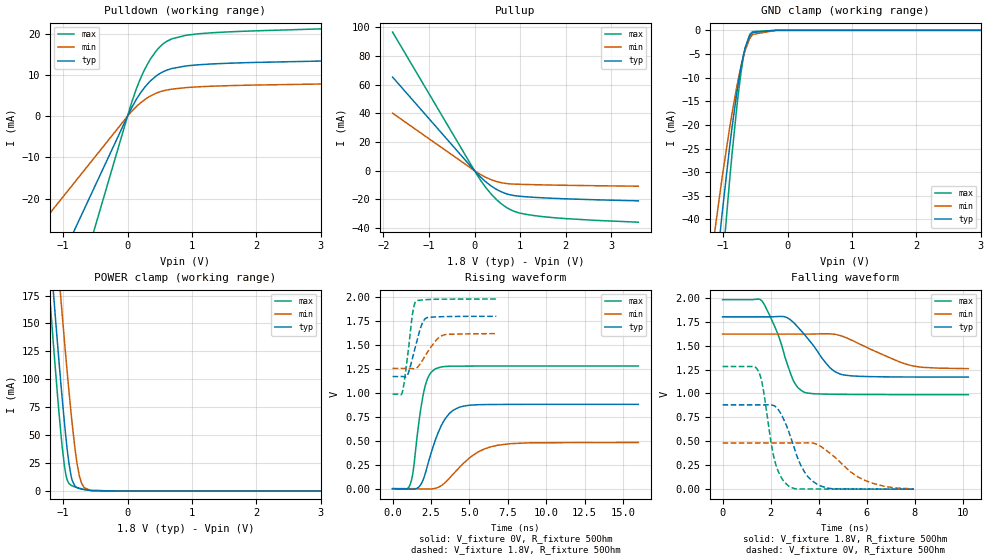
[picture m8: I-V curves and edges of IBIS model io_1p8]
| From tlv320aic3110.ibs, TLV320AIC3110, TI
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|   io_1p8 Model
[Model]   io_1p8
Model_type   I/O
Polarity   Non-Inverting
Enable   Active-High
Vinl = 0.54
Vinh = 1.26
Vmeas = 0.9
Vref = 0
Cref = 10pF
Rref = 100
|   typ   min   max
|   (nom PVT)   (fast PVT)   (slow PVT)
C_comp   1.467e-12   1.439e-12   1.494e-12
| Where nom  PVT is Nominal Process, 1.8V, 27C
|   Fast PVT is Strong Process,  1.98V, -40C
|   Slow PVT is Weak Process,   1.62V, 125C
[Model spec]
Vinl   0.54   0.486   0.594
Vinh   1.26   1.134   1.386
[Voltage Range]   1.8   1.62   1.98
|Junction Temperature
[Temperature Range]   27   125   -40
[Pullup Reference]   1.8   1.62   1.98
[Pulldown Reference]   0   0   0
[Power Clamp Reference]   1.8   1.62   1.98
[GND Clamp Reference]   0   0   0
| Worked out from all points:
|   slope of the pulldown table from 0 to 0.27 V, typ, clamps not added: 38.1 ohm
|   slope of the pullup table from 0 to 0.27 V, typ, clamps not added: 32.3 ohm
|   GND clamp passes 1 mA (typ) near -0.58 V on its own axis
|   POWER clamp passes 1 mA (typ) near -0.65 V on its own axis
|   falling waveform, V_fixture 1.8V, R_fixture 50Ohm: 20-80 % time 1.17ns typ, 1.9ns min, 842ps max; typ from 1.8 V to 1.17 V
|   rising waveform, V_fixture 0V, R_fixture 50Ohm: 20-80 % time 1.17ns typ, 1.99ns min, 651ps max; typ from 0 V to 0.881 V
|   rising waveform, V_fixture 1.8V, R_fixture 50Ohm: 20-80 % time 624ps typ, 920ps min, 442ps max; typ from 1.17 V to 1.8 V
|   falling waveform, V_fixture 0V, R_fixture 50Ohm: 20-80 % time 831ps typ, 1.46ns min, 513ps max; typ from 0.881 V to 0 V
[Pulldown]
|   Voltage   I(typ)   I(min)   I(max)
-1.8V     -60.44mA   -35.18mA   -96.09mA
-85.32mV  -2.865mA   -1.668mA   -4.555mA
67.86mV   2.164mA    1.237mA    3.517mA
173.2mV   5mA        2.868mA    8.101mA
252.5mV   6.752mA    3.877mA    10.93mA
356.2mV   8.586mA    4.927mA    13.91mA
443.3mV   9.762mA    5.588mA    15.84mA
605.7mV   11.18mA    6.359mA    18.17mA
688.9mV   11.6mA     6.589mA    18.81mA
898.9mV   12.2mA     6.948mA    19.65mA
1.307V    12.71mA    7.299mA    20.29mA
3.598V    13.69mA    8.018mA    21.69mA
[GND Clamp]
|   Voltage   I(typ)   I(min)   I(max)
-1.8V     -228.8mA   -131.4mA   -346.6mA
-1.18V    -60.79mA   -47.45mA   -78.73mA
-1.018V   -38.93mA   -31.27mA   -50.57mA
-898.2mV  -24.52mA   -20.52mA   -31.5mA
-783mV    -12.73mA   -11.53mA   -15.61mA
-736.7mV  -8.832mA   -8.46mA    -10.36mA
-685.8mV  -5.288mA   -5.563mA   -5.688mA
-657.5mV  -3.723mA   -4.215mA   -3.718mA
-588.2mV  -1.211mA   -1.797mA   -915uA
-541.8mV  -455.1uA   -870.4uA   -271.3uA
-180mV    0A         -194.6nA   0A
3.598V    0A         0A         0A
[Pullup]
|   Voltage   I(typ)   I(min)   I(max)
-1.8V     65.35mA    40.15mA    96.77mA
67.14mV   -2.325mA   -1.411mA   -3.476mA
207.7mV   -6.661mA   -3.989mA   -10.05mA
360mV     -10.54mA   -6.205mA   -16.11mA
591.8mV   -14.82mA   -8.42mA    -23.2mA
720.7mV   -16.34mA   -9.058mA   -26.04mA
898.9mV   -17.53mA   -9.423mA   -28.71mA
1.331V    -18.66mA   -9.804mA   -31.46mA
1.981V    -19.63mA   -10.2mA    -33.43mA
3.598V    -21.07mA   -10.85mA   -35.98mA
[POWER Clamp]
|   Voltage   I(typ)   I(min)   I(max)
-1.8V     683mA      751.1mA    650.3mA
-1.215V   224.9mA    301.8mA    179.4mA
-1.184V   202.1mA    279.2mA    156.2mA
-1.137V   167.6mA    244.9mA    121.2mA
-1.032V   94.01mA    170mA      49.48mA
-959.4mV  49.04mA    120.9mA    15.03mA
-876.6mV  13.34mA    69.64mA    5.038mA
-816.7mV  4.338mA    38.31mA    3.606mA
-747mV    2.078mA    13.26mA    2.384mA
-674.1mV  1.18mA     3.013mA    1.351mA
-578.3mV  431.7uA    544.6uA    424.2uA
3.598V    0A         0A         0A
[Ramp]
R_load = 50
|   typ   min   max
dV/dt_r   0.52844/1.16363e-09   0.289575/1.9791e-09   0.768595/6.51078e-10
dV/dt_f   0.377553/1.16602e-09   0.217999/1.91494e-09   0.595446/8.39797e-10
[Falling Waveform]
V_fixture = 1.8V
V_fixture_min = 1.62V
V_fixture_max = 1.98V
R_fixture = 50Ohm
|   Time   V(typ)   V(min)   V(max)
0s        1.8V       1.62V      1.98V
1.634ns   1.8V       1.62V      1.968V
2.288ns   1.804V     1.62V      1.629V
2.672ns   1.794V     1.62V      1.323V
2.927ns   1.747V     1.62V      1.145V
3.383ns   1.623V     1.62V      1.015V
4.456ns   1.272V     1.623V     992mV
4.941ns   1.199V     1.601V     990.4mV
7.836ns   1.172V     1.292V     987.8mV
10.23ns   1.171V     1.259V     987.6mV
[Rising Waveform]
V_fixture = 0V
V_fixture_min = 0V
V_fixture_max = 0V
R_fixture = 50Ohm
|   Time   V(typ)   V(min)   V(max)
0s        982.6pV    22.07nV    579.6pV
1.163ns   -4.767mV   75.04uV    51.74mV
1.352ns   -5.16mV    326.5uV    193.8mV
1.754ns   25.18mV    -2.679mV   741.6mV
2.05ns    117.8mV    -3.762mV   1.024V
2.802ns   514.5mV    4.754mV    1.252V
3.984ns   822.4mV    158.7mV    1.279V
5.239ns   874mV      349.2mV    1.28V
6.822ns   879.4mV    452.9mV    1.281V
16ns      880.7mV    482.6mV    1.281V
[Rising Waveform]
V_fixture = 1.8V
V_fixture_min = 1.62V
V_fixture_max = 1.98V
R_fixture = 50Ohm
|   Time   V(typ)   V(min)   V(max)
0s        1.171V     1.257V     987.6mV
643ps     1.171V     1.257V     1.011V
949ps     1.179V     1.257V     1.346V
1.308ns   1.371V     1.254V     1.835V
1.55ns    1.52V      1.258V     1.961V
1.963ns   1.736V     1.345V     1.971V
2.283ns   1.788V     1.428V     1.975V
2.905ns   1.794V     1.563V     1.978V
3.379ns   1.797V     1.607V     1.979V
6.754ns   1.8V       1.619V     1.98V
[Falling Waveform]
V_fixture = 0V
V_fixture_min = 0V
V_fixture_max = 0V
R_fixture = 50Ohm
|   Time   V(typ)   V(min)   V(max)
0s        880.7mV    482.7mV    1.281V
1.47ns    880.7mV    482.7mV    1.243V
1.677ns   880.7mV    482.7mV    1.067V
2.164ns   869.7mV    482.7mV    304.7mV
2.432ns   785.6mV    482.7mV    127.3mV
2.777ns   585.8mV    482.7mV    27.8mV
3.398ns   185.3mV    483.1mV    1.387mV
4.005ns   41.98mV    458.8mV    1.375mV
5.924ns   1.17mV     91.68mV    331uV
7.965ns   307.4uV    2.159mV    86.78uV
